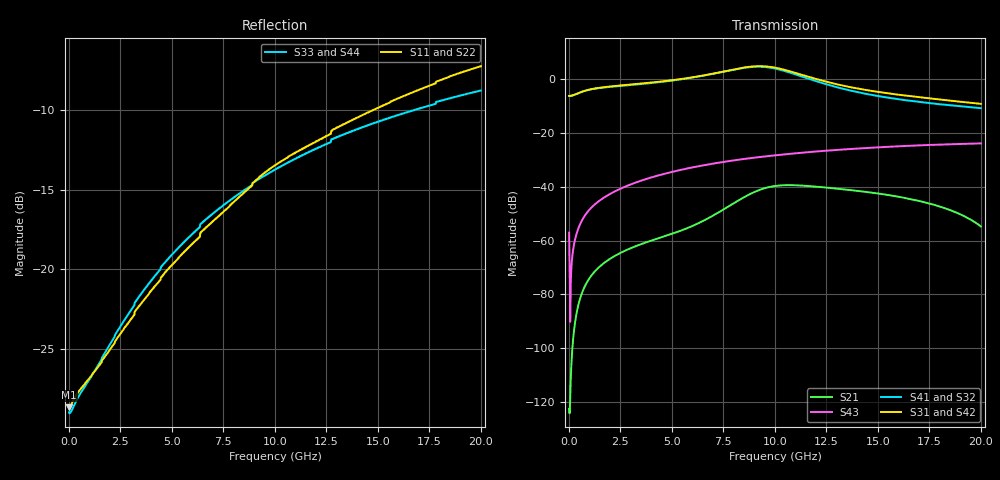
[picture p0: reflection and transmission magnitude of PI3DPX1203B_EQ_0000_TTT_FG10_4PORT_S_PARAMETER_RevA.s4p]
! NPort=4 DATA=2000 NOISE=0 GROUPDELAY=0 COMPLEX_DATAFORMAT=POLAR
! NumOfBlock=1 NumOfParam=0
! .MODEL Smodel S TSTONEFILE=PI3DPX1203B_EQ_0000_TTT_FG10_4PORT_S_PARAMETER_RevA.s4p TYPE=S
!  -- The above .MODEL line can be used for the S element in the netlist.
! The s parameter is extracted from the linear redriver, it is not bi-directional; only s(4,1)s(4,2) and s(3,1)s(3,2)
! should be the insertion loss
!Port definition:
!Port1 = input+
!Port2 = input-
!Port3 = output+
!Port4 = output-
# Hz S MA R  50
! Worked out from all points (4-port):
!   2000 points, 10 MHz to 20 GHz, reference 50 ohm
!   strongest paths, dB at 10 MHz, 5.01 GHz, 10.01 GHz, 15.01 GHz, 20 GHz:
!     S31: -6.2, -0.3, 4.4, -4.7, -9.1
!     S42: -6.2, -0.3, 4.4, -4.7, -9.1
!     S41: -6.2, -0.4, 4.0, -6.2, -10.7
!     S32: -6.2, -0.4, 4.0, -6.2, -10.7
!     S43: -57.1, -34.4, -28.3, -25.3, -23.8
!     S21: -122.7, -57.5, -39.7, -42.5, -54.8
!   lowest |S11| = -28.6 dB at 10 MHz (marker M1), VSWR 1.08, Z = 46.4 - j0.0306 ohm
!   |S11| at or under -10 dB: start of sweep to 14.77 GHz
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1e7  0.03701 -179.5  7.338e-07 10.5  0 0.0  0 0.0
     7.338e-07 10.5  0.03701 -179.5  0 0.0  0 0.0
     0.4917 -0.2  0.4917 179.8  0.03566 178.2  0.001403 -77.8
     0.4917 179.8  0.4917 -0.2  0.001403 -77.8  0.03566 178.2
1.57e9  0.05097 -144.8  0.0003463 112.4  5.226e-12 74.9  4.902e-11 115.4
        0.0003463 112.4  0.05097 -144.8  4.902e-11 115.4  5.226e-12 74.9
        0.7045 -2.5  0.6981 177.4  0.05202 -142.1  0.005823 82.8
        0.6981 177.4  0.7045 -2.5  0.005823 82.8  0.05202 -142.1
6.13e9  0.1226 -111.7  0.001968 113.8  1.442e-08 -103.1  1.481e-07 67.7
        0.001967 113.8  0.1226 -111.7  1.48e-07 67.7  1.442e-08 -103.0
        1.113 -52.5  1.103 130.3  0.1317 -116.9  0.02351 64.5
        1.103 130.4  1.113 -52.5  0.02351 64.5  0.1317 -116.9
8.71e9  0.179 -106.7  0.007064 96.7  4.372e-07 162.2  1.259e-06 16.8
        0.007061 96.7  0.179 -106.7  1.258e-06 16.9  4.373e-07 162.3
        1.707 -103.2  1.677 79.2  0.1805 -115.9  0.03379 51.3
        1.679 79.2  1.706 -103.3  0.03379 51.3  0.1805 -115.9
1.016e10  0.2153 -107.5  0.01052 56.0  1.384e-06 98.7  2.472e-06 -21.5
          0.01052 56.1  0.2153 -107.5  2.468e-06 -21.4  1.384e-06 98.7
          1.609 -148.8  1.542 33.4  0.208 -116.4  0.03906 43.5
          1.544 33.4  1.607 -148.8  0.03906 43.5  0.208 -116.4
1.224e10  0.2562 -108.5  0.009885 11.3  3.213e-06 32.5  4.291e-06 -50.0
          0.009881 11.4  0.2562 -108.5  4.291e-06 -49.8  3.215e-06 32.5
          0.9608 169.1  0.8674 -7.6  0.2426 -117.6  0.04622 33.0
          0.8687 -7.7  0.9598 169.2  0.04622 33.0  0.2426 -117.6
2e10  0.4336 -116.1  0.001824 -80.9  2.16e-05 -105.3  3.303e-05 -134.2
      0.001826 -80.4  0.4337 -116.1  3.313e-05 -134.2  2.164e-05 -105.3
      0.3504 90.2  0.2918 -67.3  0.3637 -123.9  0.06431 -7.0
      0.2911 -67.5  0.3511 90.3  0.06431 -7.0  0.3637 -123.9
